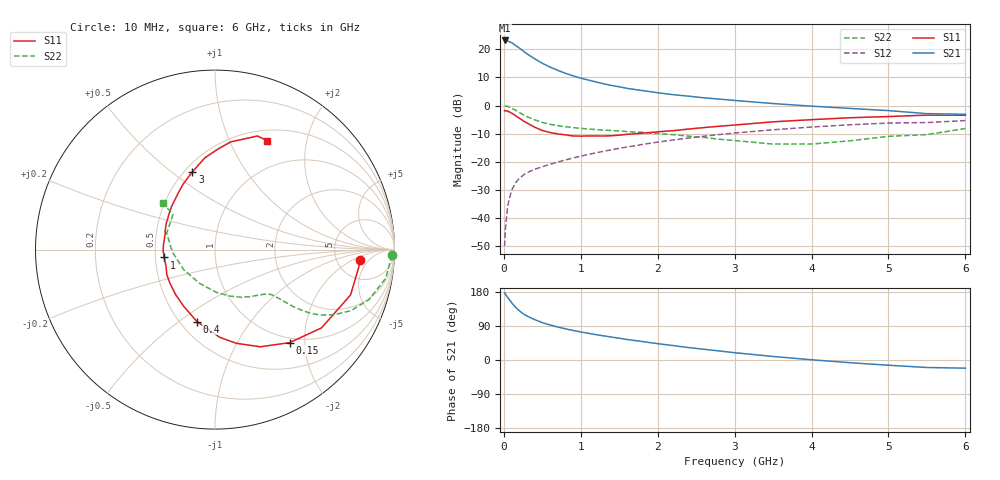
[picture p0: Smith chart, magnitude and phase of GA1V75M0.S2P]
! Infineon Technologies  Discrete & RF Semiconductors
! BF775
! Si NPN RF Bipolar Junction Transistor in SOT23
! VCE = 1.75 V  IC = 5 mA
! Common Emitter S-Parameters:  May  1996
# GHz  S  MA  R  50
!  f  S11  S21  S12  S22
! GHz  MAG  ANG  MAG  ANG  MAG  ANG  MAG  ANG
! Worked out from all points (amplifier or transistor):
!   36 points, 10 MHz to 6 GHz, reference 50 ohm
!   highest |S21| = 23.1 dB at 10 MHz (marker M1)
!   |S21| within 3 dB of that: start of sweep to 216.7 MHz
!   unconditionally stable (mu >= 1): 757.1 MHz to 4.147 GHz; 5.193 GHz to end of sweep
!   at 250 MHz: K = 0.50, MSG = 22.1 dB, |S12| = -24.7 dB
!   at 1.4 GHz: K = 1.15, MAG = 9.0 dB, |S12| = -15.7 dB
!   at 6 GHz: K = 1.00, MAG = 0.9 dB, |S12| = -5.3 dB
!   S11 on the Smith chart (normalised r, x): 10 MHz: 8.73, -2.84; 150 MHz: 0.92, -1.70; 400 MHz: 0.60, -0.58; 1 GHz: 0.56, -0.05; 3 GHz: 0.55, +0.60; 6 GHz: 0.63, +1.40
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0.01  0.8125 -3.9  14.26 177.1  0.0032 87.6  0.9889 -1.9
0.02  0.8057 -7.6  14.01 173.8  0.0064 87.3  0.9787 -3.8
0.05  0.7963 -18.5  13.9 165.3  0.0167 80.6  0.965 -9.5
0.1  0.7367 -36.3  13.08 151.8  0.031 72.4  0.9028 -17.9
0.15  0.6643 -51.3  11.67 139.7  0.0422 64.5  0.8299 -24.2
0.2  0.5974 -65.0  10.51 130.3  0.0509 60.7  0.7557 -28.7
0.25  0.5356 -77.1  9.322 122.2  0.0579 57.5  0.6874 -32.0
0.3  0.49 -86.8  8.266 116.2  0.0644 55.8  0.6362 -33.8
0.4  0.4131 -104.1  6.753 106.6  0.0737 53.5  0.5573 -35.8
0.5  0.3612 -118.8  5.608 98.5  0.0822 53.3  0.5012 -36.6
0.6  0.3327 -131.4  4.822 92.4  0.0906 53.9  0.4645 -37.1
0.8  0.3022 -152.8  3.727 82.3  0.1081 54.2  0.4207 -38.0
1  0.2865 -171.2  3.066 74.1  0.1263 55.1  0.3937 -39.2
1.1  0.2891 -178.7  2.824 70.4  0.1357 55.3  0.3832 -40.5
1.3  0.288 168.3  2.426 63.6  0.1546 54.8  0.3663 -42.8
1.6  0.3082 151.9  2.019 54.2  0.1838 53.7  0.3456 -47.6
2.2  0.3577 128.4  1.557 38.1  0.2445 49.3  0.3047 -60.7
3  0.4509 106.2  1.231 19.3  0.3253 40.8  0.239 -87.9
3.5  0.5139 96.4  1.084 9.3  0.3715 34.5  0.2071 -114.4
4.5  0.607 81.6  0.888 -7.1  0.4557 21.3  0.2368 -176.1
5.5  0.6758 69.5  0.718 -19.8  0.4987 6.8  0.3048 140.3
6  0.673 64.3  0.699 -21.6  0.5405 2.8  0.3914 137.9
